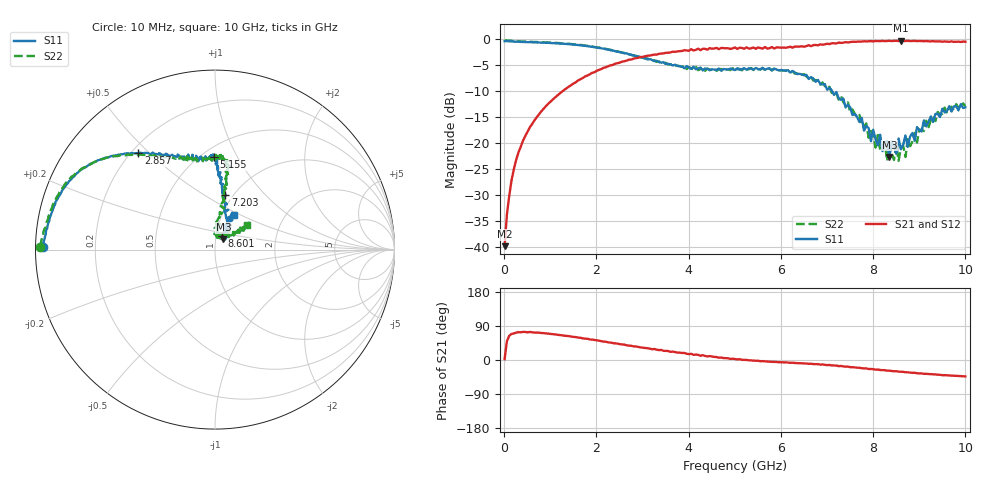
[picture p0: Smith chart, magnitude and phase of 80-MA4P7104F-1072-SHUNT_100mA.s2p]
!Agilent Technologies,E8364C,MY48140145,A.09.42.15
!Agilent E8364C: A.09.42.15
!Date: Wednesday, December 02, 2020 11:09:13
!Correction: S11(Full 2 Port(1,2))
!S21(Full 2 Port(1,2))
!S12(Full 2 Port(1,2))
!S22(Full 2 Port(1,2))
!S2P File: Measurements: S11, S21, S12, S22:
# Hz S  dB  R 50
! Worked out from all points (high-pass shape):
!   201 points, 10 MHz to 10 GHz, reference 50 ohm
!   highest |S21| = -0.30 dB at 8.601 GHz (marker M1); lowest = -39.9 dB at 10 MHz (marker M2)
!   |S21| within 3 dB of the highest: 3.054 GHz to end of sweep
!   lowest |S11| = -22.7 dB at 8.352 GHz (marker M3), VSWR 1.16, Z = 54.5 + j6.2 ohm
!   |S11| at or under -10 dB: 7.111 GHz to end of sweep
!   |S22| runs from -23.4 to -0.2 dB; largest |S21 - S12| = 0.032
!   S11 on the Smith chart (normalised r, x): 10 MHz: 0.02, +0.01; 2.857 GHz: 0.23, +0.46; 5.155 GHz: 0.58, +0.81; 7.203 GHz: 0.92, +0.62; 8.601 GHz: 1.07, +0.17; 10 GHz: 1.14, +0.46
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1e7  -0.37 179.0  -39.89 2.1  -45.93 17.3  -0.23 179.1
5.995e7  -0.37 178.6  -33.80 49.7  -33.97 49.5  -0.23 178.4
1.099e8  -0.40 177.4  -30.23 63.9  -29.99 63.1  -0.28 177.1
3.5965e8  -0.51 172.9  -20.73 73.0  -20.68 73.0  -0.44 172.4
8.5915e8  -0.67 164.2  -13.36 70.9  -13.35 70.8  -0.58 163.8
1.7083e9  -1.20 149.5  -7.45 57.0  -7.40 57.4  -1.16 149.9
2.85715e9  -3.26 128.5  -3.64 35.7  -3.68 35.2  -3.18 130.1
3.35665e9  -4.41 119.0  -2.81 26.1  -2.90 26.8  -4.28 120.7
5.005e9  -5.94 91.1  -1.57 2.6  -1.50 1.8  -6.10 91.9
5.15485e9  -5.78 90.7  -1.67 0.7  -1.59 0.5  -5.99 89.3
6.7033e9  -7.57 87.6  -1.13 -10.9  -1.08 -10.0  -7.97 81.7
7.2028e9  -10.18 79.2  -0.82 -14.8  -0.79 -15.3  -10.43 81.9
8.05195e9  -19.34 63.8  -0.33 -25.3  -0.34 -24.7  -20.87 80.2
8.25175e9  -20.23 41.3  -0.37 -26.8  -0.35 -27.4  -19.80 86.8
8.3017e9  -19.62 55.8  -0.33 -28.2  -0.28 -27.4  -23.44 81.7
8.35165e9  -22.69 50.4  -0.30 -28.2  -0.34 -28.7  -20.48 71.7
8.4016e9  -19.69 42.9  -0.35 -28.9  -0.29 -29.1  -21.69 87.3
8.6014e9  -21.20 62.3  -0.30 -31.1  -0.34 -31.0  -20.95 55.0
8.7013e9  -18.55 57.8  -0.33 -32.5  -0.28 -31.6  -22.69 53.1
8.75125e9  -20.75 60.5  -0.30 -32.5  -0.34 -32.9  -19.26 52.3
9.1009e9  -15.64 61.8  -0.38 -36.5  -0.32 -35.6  -17.69 36.9
1e10  -13.12 61.1  -0.48 -43.2  -0.48 -43.4  -12.88 37.6
